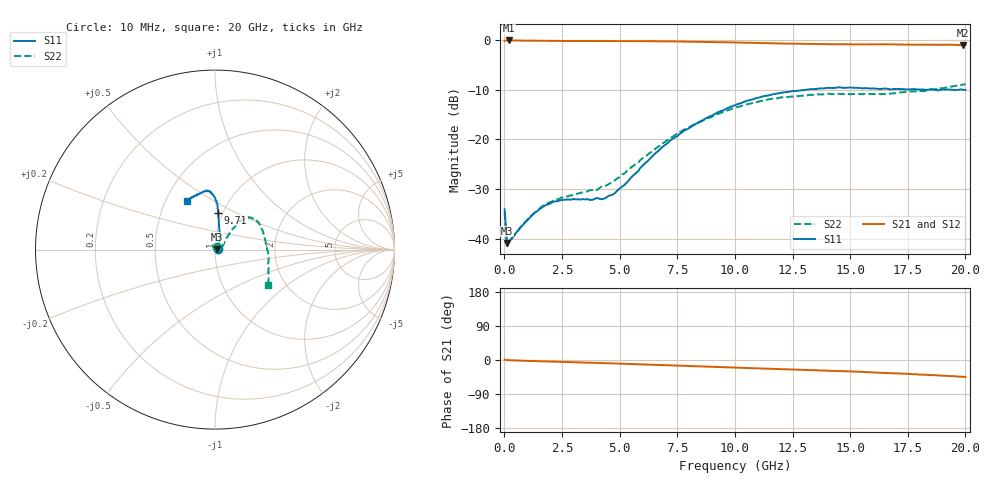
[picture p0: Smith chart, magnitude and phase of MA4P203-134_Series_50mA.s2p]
! AWR Design Environment (9226) Thu Aug 19 14:29:25 2021
! Document = '50mA'
! nPorts: 2, nXvals: 201
# GHz S DB R 50
!Freq DBS11 AngS11 DBS21 AngS21 DBS12 AngS12 DBS22 AngS22
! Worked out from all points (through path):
!   201 points, 10 MHz to 20 GHz, reference 50 ohm
!   highest |S21| = -0.13 dB at 210 MHz (marker M1); lowest = -1.1 dB at 19.91 GHz (marker M2)
!   group delay of S21, straight-line fit = 5.93 ps
!   lowest |S11| = -40.9 dB at 110 MHz (marker M3), VSWR 1.02, Z = 50.9 + j0.0581 ohm
!   |S11| at or under -10 dB: start of sweep to 13.16 GHz; 18.16 GHz to 18.44 GHz (270.9 MHz wide, 1.48 % of centre); 19.33 GHz to 19.78 GHz (451.1 MHz wide, 2.31 % of centre)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
!   |S22| runs from -41.5 to -8.9 dB; largest |S21 - S12| = 0.043
!   S11 on the Smith chart (normalised r, x): 10 MHz: 1.04, +0.01; 9.71 GHz: 0.95, +0.41; 20 GHz: 0.64, +0.38
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0.01  -34.06 16.6  -0.20 1.0  -0.17 0.7  -34.74 41.0
0.11  -40.87 3.6  -0.13 -0.3  -0.12 -0.3  -41.49 2.8
0.21  -40.49 5.5  -0.13 -0.5  -0.12 -0.5  -40.56 7.8
1.21  -35.24 -4.0  -0.18 -2.7  -0.17 -2.6  -35.16 -2.5
1.81  -33.21 -13.8  -0.21 -3.8  -0.20 -3.5  -33.01 -11.6
2.41  -32.28 -19.2  -0.23 -4.8  -0.22 -4.5  -31.88 -16.6
3.41  -32.01 -12.3  -0.24 -6.6  -0.23 -6.1  -30.66 -10.4
3.81  -32.18 -3.8  -0.25 -7.3  -0.23 -6.8  -30.21 -4.3
4.01  -31.82 1.2  -0.25 -7.7  -0.23 -7.2  -30.23 0.1
4.21  -32.05 10.3  -0.25 -8.0  -0.23 -7.5  -29.52 3.5
4.71  -31.10 26.9  -0.26 -8.9  -0.24 -8.4  -28.42 13.2
6.71  -22.21 70.7  -0.30 -13.0  -0.27 -12.2  -21.38 43.5
7.81  -18.23 79.0  -0.35 -15.4  -0.35 -14.5  -18.02 48.1
9.71  -13.66 85.3  -0.51 -19.5  -0.50 -18.3  -14.13 48.9
10.01  -13.13 85.3  -0.54 -20.3  -0.53 -18.9  -13.65 48.9
11.21  -11.36 88.1  -0.65 -22.8  -0.65 -21.1  -12.23 46.0
13.41  -9.91 94.6  -0.84 -26.8  -0.80 -25.1  -11.04 35.8
14.51  -9.53 98.1  -0.91 -29.2  -0.84 -27.2  -10.86 28.6
16.71  -9.96 108.8  -0.93 -34.7  -0.85 -32.3  -10.82 4.1
18.21  -10.01 117.0  -0.98 -38.6  -0.88 -37.0  -10.31 -14.8
19.91  -10.05 121.5  -1.05 -44.2  -0.98 -43.0  -9.00 -32.9
20  -10.06 120.3  -1.05 -44.8  -0.99 -43.2  -8.92 -33.8
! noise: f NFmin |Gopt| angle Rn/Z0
0.01  0  1  0  2e-20
2.21  0  1  0  2e-20
4.41  0  1  0  2e-20
6.61  0  1  0  2e-20
8.81  0  1  0  2e-20
11.11  0  1  0  2e-20
13.31  0  1  0  2e-20
15.51  0  1  0  2e-20
17.71  0  1  0  2e-20
20  0  1  0  2e-20
